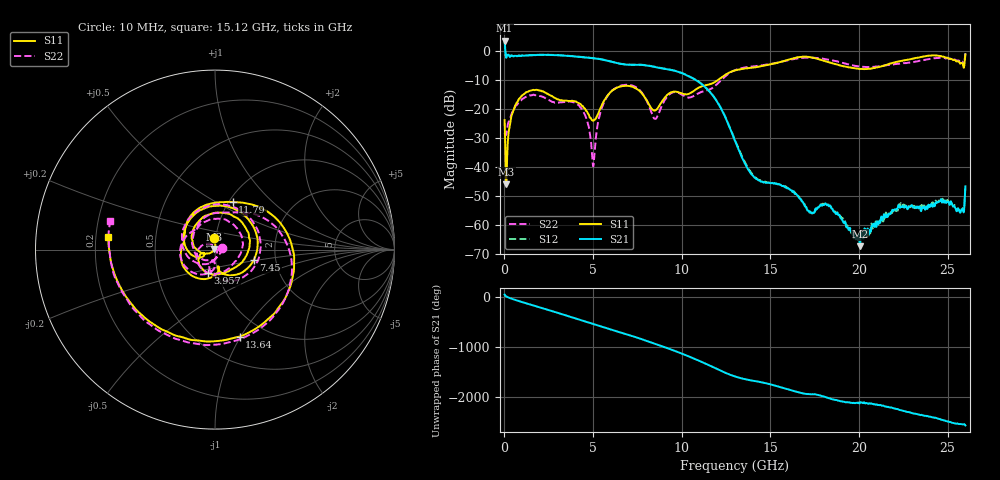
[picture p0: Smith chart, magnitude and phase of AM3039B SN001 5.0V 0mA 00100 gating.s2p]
!Agilent Technologies,E8364B,MY43040894,A.07.50.67
!Agilent E8364B: A.07.50.67
!Date: Tuesday, June 28, 2016 08:04:14
!Correction: S11(Full 2 Port(1,2))
!S21(Full 2 Port(1,2))
!S12(Full 2 Port(1,2))
!S22(Full 2 Port(1,2))
!S2P File: Measurements: S11, S21, S12, S22:
# Hz S  dB  R 50
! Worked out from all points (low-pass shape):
!   1601 points, 10 MHz to 26 GHz, reference 50 ohm
!   highest |S21| = 3.57 dB at 10 MHz (marker M1); lowest = -67.2 dB at 20.05 GHz (marker M2)
!   |S21| within 3 dB of the highest: start of sweep to 44.69 MHz
!   lowest |S11| = -46.0 dB at 107.5 MHz (marker M3), VSWR 1.01, Z = 49.5 + j0.212 ohm
!   |S11| at or under -10 dB: start of sweep to 12.05 GHz
!   |S22| runs from -39.7 to -0.8 dB; largest |S21 - S12| = 0.025
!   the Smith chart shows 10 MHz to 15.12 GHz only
!   S11 on the Smith chart (normalised r, x): 10 MHz: 0.98, +0.13; 3.957 GHz: 0.89, -0.24; 7.45 GHz: 1.54, -0.19; 11.79 GHz: 1.04, +0.60; 13.64 GHz: 0.76, -0.99; 15.12 GHz: 0.25, +0.06
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1e7  -23.80 96.9  3.57 40.5  3.63 41.4  -28.30 15.3
1.074625e8  -45.96 154.8  -2.31 3.3  -2.24 3.3  -28.69 -60.7
7.572125e8  -17.26 157.3  -1.69 -82.7  -1.65 -82.5  -18.09 172.5
1.618131e9  -13.40 68.7  -1.41 -174.9  -1.37 -174.8  -15.07 73.2
2.609e9  -15.38 -19.3  -1.35 79.8  -1.30 79.9  -17.25 -17.7
3.957231e9  -17.32 -107.6  -1.90 -65.9  -1.82 -65.6  -17.74 -125.6
4.347081e9  -18.73 -140.4  -2.11 -108.5  -2.07 -108.3  -19.84 -169.5
5.013075e9  -24.04 -158.1  -2.51 178.0  -2.45 178.4  -39.74 16.8
5.7278e9  -16.11 179.7  -3.24 96.9  -3.17 97.4  -16.35 -162.3
7.449638e9  -12.98 -14.9  -4.75 -91.4  -4.70 -90.9  -12.59 -29.9
8.684162e9  -19.34 -77.7  -5.76 119.5  -5.69 120.2  -21.82 -90.0
1.178672e10  -10.98 69.6  -15.60 37.1  -15.50 38.5  -12.53 61.5
1.3005e10  -6.70 -22.3  -30.96 -146.5  -30.65 -144.4  -6.60 -28.8
1.363851e10  -5.96 -74.2  -39.61 154.6  -39.23 155.6  -5.62 -82.5
1.511669e10  -4.47 173.0  -45.45 45.9  -45.43 46.4  -4.36 165.0
1.630248e10  -2.51 74.9  -48.30 -71.6  -48.51 -70.8  -2.80 72.4
1.734208e10  -2.25 -24.8  -55.87 -138.7  -55.83 -140.3  -2.30 -16.5
2.005479e10  -6.20 120.2  -67.23 54.0  -62.76 47.0  -5.37 130.0
2.167916e10  -4.46 12.4  -56.02 -35.2  -55.86 -36.2  -4.84 18.0
2.309237e10  -2.59 -93.6  -53.94 -160.5  -53.29 -160.4  -3.77 -84.0
2.41807e10  -1.52 178.1  -53.06 122.9  -52.25 116.9  -2.52 -167.1
2.6e10  -1.24 -25.4  -46.63 -38.7  -46.33 -38.7  -0.76 2.4
